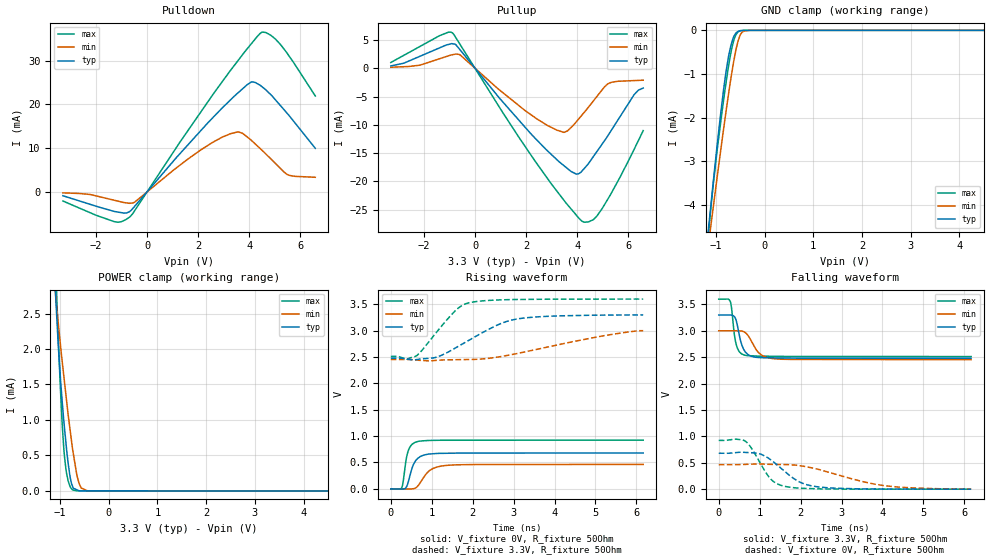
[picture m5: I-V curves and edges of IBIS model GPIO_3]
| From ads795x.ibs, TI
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|   Output GPIO model 3V
[Model]   GPIO_3
Model_type   I/O
|Signals   GPIO0, GPIO1, GPIO2, GPIO3
Vinl = 0.4
Vinh = 2.31
Vmeas = 1.65
Vref = 1.65
Cref = 15pF
Rref = 50
| variable   typ   min   max
|C_comp Input mode
C_comp   1.0953352e-12   1.3398109e-12   8.6296588e-13
|C_comp Output High
|C_comp   8.1003045e-11   2.9667704e-11   1.7378310e-10
|C_comp Output Low
|C_comp   3.4569429e-11   1.3879844e-11   8.1545936e-11
|   typ   min   max
[Voltage Range]   3.3   3   3.6
[Temperature Range]   27   125   -40
[Pullup Reference]   3.3   3   3.6
[Pulldown Reference]   0   0   0
[Power Clamp Reference]   3.3   3   3.6
[GND Clamp Reference]   0   0   0
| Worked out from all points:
|   slope of the pulldown table from 0 to 0.495 V, typ, clamps not added: 147 ohm
|   slope of the pullup table from 0 to 0.495 V, typ, clamps not added: 181 ohm
|   GND clamp passes 1 mA (typ) near -0.80 V on its own axis
|   POWER clamp passes 1 mA (typ) near -0.92 V on its own axis
|   falling waveform, V_fixture 3.3V, R_fixture 50Ohm: 20-80 % time 168ps typ, 276ps min, 112ps max; typ from 3.3 V to 2.48 V
|   rising waveform, V_fixture 0V, R_fixture 50Ohm: 20-80 % time 190ps typ, 299ps min, 125ps max; typ from 0 V to 0.681 V
|   rising waveform, V_fixture 3.3V, R_fixture 50Ohm: 20-80 % time 1.18ns typ, 2.04ns min, 714ps max; typ from 2.48 V to 3.3 V
|   falling waveform, V_fixture 0V, R_fixture 50Ohm: 20-80 % time 686ps typ, 1.38ns min, 449ps max; typ from 0.681 V to 0 V
[Pulldown]
|   Voltage   I(typ)   I(min)   I(max)
-3.3V     -901.2uA   -242.5uA   -2.105mA
-1.297V   -4.478mA   -1.923mA   -6.817mA
-687.2mV  -4.528mA   -2.631mA   -5.799mA
-483mV    -3.29mA    -2.353mA   -4.281mA
2.101V    13.99mA    9.583mA    18.25mA
3.268V    21.05mA    13.31mA    27.81mA
3.566V    22.69mA    13.73mA    30.09mA
4.093V    25.18mA    11.74mA    33.97mA
4.496V    24.09mA    9.551mA    36.54mA
5.024V    21.09mA    6.515mA    35.01mA
5.496V    17.93mA    3.948mA    31.66mA
6.59V     9.958mA    3.325mA    21.95mA
[GND Clamp]
|   Voltage   I(typ)   I(min)   I(max)
-3.3V     -29.63mA   -24.44mA   -36.26mA
-1.156V   -4.593mA   -4.945mA   -4.719mA
-1.099V   -3.972mA   -4.445mA   -4.037mA
-970.4mV  -2.603mA   -3.339mA   -2.72mA
-842.4mV  -1.371mA   -2.272mA   -1.611mA
-787.1mV  -920.1uA   -1.826mA   -1.173mA
-733.7mV  -564.6uA   -1.417mA   -784.7uA
-663.5mV  -245.7uA   -912.9uA   -366.2uA
-551.3mV  -27.46uA   -277.2uA   -44.54uA
-461.8mV  -4.538uA   -44.74uA   -5.314uA
-306.3mV  -771.1nA   -596nA     -732.3nA
6.59V     0A         0A         0A
[Pullup]
|   Voltage   I(typ)   I(min)   I(max)
-3.3V     432.2uA    202.9uA    1.045mA
-889.9mV  4.367mA    2.415mA    6.29mA
-573.8mV  3.213mA    2.351mA    4.148mA
1.961V    -10.4mA    -7.464mA   -13.8mA
3.209V    -16.16mA   -10.93mA   -21.72mA
3.63V     -17.75mA   -11.04mA   -24.16mA
3.97V     -18.71mA   -9.44mA    -25.98mA
4.266V    -17.78mA   -7.85mA    -27.21mA
4.64V     -15.58mA   -5.741mA   -26.75mA
5.205V    -11.91mA   -2.721mA   -23.12mA
6.234V    -4.649mA   -2.156mA   -14.32mA
6.59V     -3.471mA   -2.087mA   -11.02mA
[POWER Clamp]
|   Voltage   I(typ)   I(min)   I(max)
-3.3V     43.35mA    34.07mA    53.59mA
-1.089V   2.732mA    2.748mA    3.144mA
-1.072V   2.513mA    2.613mA    2.825mA
-1.064V   2.418mA    2.558mA    2.687mA
-997.2mV  1.646mA    2.099mA    1.518mA
-961.8mV  1.318mA    1.864mA    1.021mA
-916.2mV  944.1uA    1.583mA    549uA
-834.9mV  401.1uA    1.085mA    145.8uA
-745.3mV  69.42uA    604.3uA    16.03uA
-609mV    2.205uA    106.3uA    1.305uA
-434.3mV  936.7nA    1.154uA    1.273uA
6.59V     0A         0A         0A
[Ramp]
R_load = 50
|   typ   min   max
dV/dt_r   0.408362/1.88831e-010  0.278215/2.9439e-010   0.554434/1.24286e-010
dV/dt_f   0.49235/1.66977e-010  0.327672/2.73553e-010  0.652452/1.11541e-010
[Falling Waveform]
V_fixture = 3.3V
V_fixture_min = 3V
V_fixture_max = 3.6V
R_fixture = 50Ohm
C_fixture = 0F
|   Time   V(typ)   V(min)   V(max)
0s        3.3V       3V         3.6V
278.2ps   3.301V     3V         3.564V
315.7ps   3.298V     3V         3.415V
383.7ps   3.269V     3.001V     2.922V
429ps     3.188V     3.001V     2.739V
537.9ps   2.798V     2.998V     2.578V
635.2ps   2.618V     2.973V     2.539V
988.6ps   2.494V     2.576V     2.521V
1.332ns   2.488V     2.472V     2.518V
6.166ns   2.479V     2.454V     2.513V
[Rising Waveform]
V_fixture = 0V
V_fixture_min = 0V
V_fixture_max = 0V
R_fixture = 50Ohm
C_fixture = 0F
|   Time   V(typ)   V(min)   V(max)
0s        -282.1nV   -343.1nV   -214.1nV
262.9ps   -2.601mV   -962.6uV   17.01mV
299.6ps   -2.964mV   -1.097mV   127.5mV
363.3ps   16.25mV    -1.33mV    496.7mV
429ps     139.7mV    -1.571mV   727.5mV
557.5ps   469.6mV    3.081mV    865.5mV
672.5ps   585.9mV    65.46mV    900.7mV
956.5ps   661.8mV    352.6mV    918.5mV
1.363ns   674.8mV    445.3mV    921.9mV
6.166ns   680.6mV    463.7mV    924.1mV
[Rising Waveform]
V_fixture = 3.3V
V_fixture_min = 3V
V_fixture_max = 3.6V
R_fixture = 50Ohm
C_fixture = 0F
|   Time   V(typ)   V(min)   V(max)
0s        2.479V     2.454V     2.513V
390.7ps   2.462V     2.454V     2.459V
630.4ps   2.452V     2.443V     2.526V
1.127ns   2.5V       2.439V     2.98V
1.552ns   2.661V     2.449V     3.36V
1.924ns   2.825V     2.454V     3.532V
2.68ns    3.133V     2.508V     3.584V
3.135ns   3.229V     2.575V     3.592V
5.113ns   3.295V     2.892V     3.599V
6.166ns   3.3V       3V         3.6V
[Falling Waveform]
|Gnd
V_fixture = 0V
V_fixture_min = 0V
V_fixture_max = 0V
R_fixture = 50Ohm
C_fixture = 0F
|   Time   V(typ)   V(min)   V(max)
0s        680.6mV    463.7mV    924.1mV
649.1ps   696.6mV    469.4mV    909.6mV
813.6ps   689mV      474.4mV    760.2mV
1.021ns   664.8mV    476.9mV    485.6mV
1.257ns   563.5mV    470.4mV    202.2mV
1.649ns   312.7mV    465.5mV    47.7mV
2.031ns   116.3mV    438.6mV    16.11mV
2.609ns   29.74mV    337.2mV    3.344mV
4.07ns    2.182mV    63.72mV    284.7uV
6.166ns   -282.1nV   -343.1nV   -214.1nV
